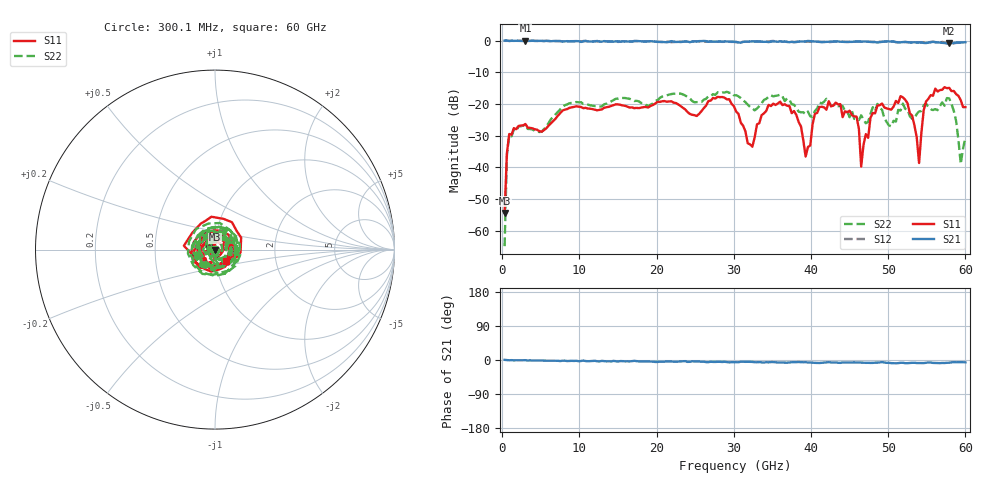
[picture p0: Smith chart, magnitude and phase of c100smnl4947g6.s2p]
! 3/17/2022 9:57:28 AM
! D:\C100SMNL4947G6.S2P
! CHANNEL.1
! TR.MEASUREMENT
! CORRECTED.DATA
# GHZ S RI R 50.0
! FREQ.GHZ  S11RE  S11IM  S21RE  S21IM  S12RE  S12IM  S22RE  S22IM
!; PortSelection: Port_12
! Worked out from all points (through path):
!   200 points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, 300.1 MHz to 60 GHz, reference 50 ohm
!   highest |S21| = 0.02 dB at 3 GHz (marker M1); lowest = -0.9 dB at 57.9 GHz (marker M2)
!   lowest |S11| = -54.4 dB at 300.1 MHz (marker M3), VSWR 1.00, Z = 49.8 + j0.0152 ohm
!   |S11| at or under -10 dB: start of sweep to end of sweep
!   |S22| runs from -64.9 to -16.1 dB; largest |S21 - S12| = 0.037
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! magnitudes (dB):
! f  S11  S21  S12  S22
! 300.1 MHz  -54.4  0.0  0.1  -64.9
! 600.1 MHz  -35.4  0.0  0.0  -35.9
! 900.1 MHz  -29.5  -0.1  -0.1  -29.9
! 3 GHz  -26.3  0.0  0.0  -26.7
! 10.5 GHz  -21.3  -0.2  -0.1  -20.0
! 20.4 GHz  -19.3  -0.4  -0.4  -18.1
! 30.3 GHz  -22.4  -0.4  -0.5  -17.2
! 32.4 GHz  -33.5  -0.2  -0.3  -21.4
! 34.5 GHz  -20.3  -0.5  -0.3  -17.7
! 37.2 GHz  -20.6  -0.5  -0.4  -18.6
! 39.3 GHz  -36.6  -0.2  -0.3  -23.2
! 40.2 GHz  -26.4  -0.2  -0.3  -24.0
! 45.9 GHz  -24.0  -0.3  -0.3  -24.7
! 46.5 GHz  -39.7  -0.3  -0.3  -23.6
! 47.7 GHz  -24.4  -0.4  -0.4  -23.2
! 50.1 GHz  -21.6  -0.3  -0.2  -26.8
! 52.5 GHz  -19.7  -0.5  -0.5  -21.7
! 54 GHz  -38.6  -0.6  -0.5  -22.4
! 54.9 GHz  -19.2  -0.8  -0.6  -19.8
! 57.9 GHz  -14.9  -0.9  -1.1  -18.2
! 59.4 GHz  -18.8  -0.6  -0.6  -38.9
! 60 GHz  -21.0  -0.5  -0.5  -30.6
